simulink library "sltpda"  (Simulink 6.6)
InitFcn:
  | disp('Welcome to sLTPDA');
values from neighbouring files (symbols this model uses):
  filter = '*'    [uipickfiles.m]
  out = char(outs{j})    [sortCmds.m]    (also in uipickfiles.m = 0)
  param = params{get(handles.paramList, 'Value')}    [loopgui.m]
  plist = [plist cellstr(p.key)]    [sltpda_control.m]
undefined symbols (not defined in the file or in its folder): ao, chirp, foo_iir, Hanning, highpass, hist, Kaiser, linear, Normal, pole, pzmodel

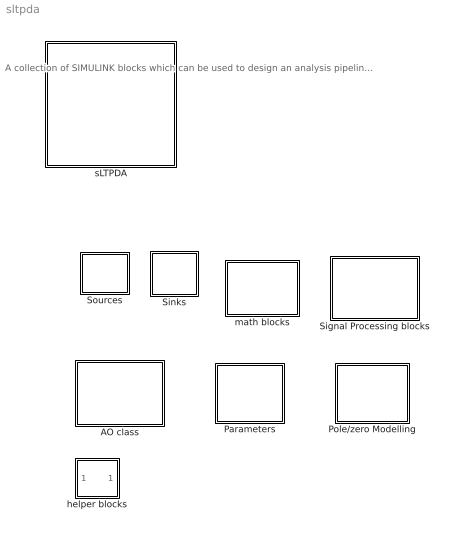
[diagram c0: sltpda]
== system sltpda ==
  note: A collection of SIMULINK blocks which can be used to design an analysis pipeline using LTPDA functions. The sLTPDA function set can be used to parse and run the model.
  AO class : Subsystem
  Parameters : Subsystem
  Pole/zero Modelling : Subsystem
  Signal Processing blocks : Subsystem
  Sinks : Subsystem
  Sources : Subsystem
  helper blocks : Subsystem
  math blocks : Subsystem
  sLTPDA : Subsystem

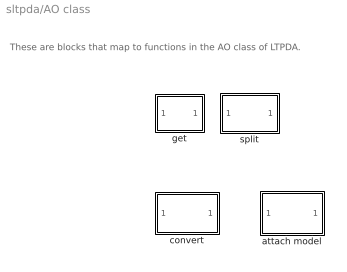
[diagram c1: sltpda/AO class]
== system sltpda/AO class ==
  note: These are blocks that map to functions in the AO class of LTPDA.
  attach model : Subsystem  Tag=attachdmdl
  convert : Subsystem  mask(convert){fcn=ao}
      mask prompts: fcn "convert to"
  get : Subsystem  Tag=get  Description=Get the propery of an analysis object.  mask(get){param=hist}
      mask prompts: param "parameter"
  split : Subsystem  Tag=split  Description=Splits an AO into many sub-AOs.  mask(split){method=times, splits=0}
      mask prompts: method "splitting method"

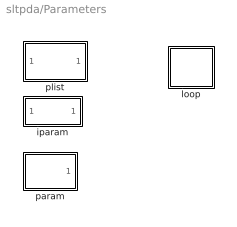
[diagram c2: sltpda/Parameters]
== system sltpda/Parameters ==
  iparam : Subsystem  Tag=iparam  mask(iparam){key=0}
      mask prompts: key "Parameter name"
  loop : Subsystem  mask(loop){block=<empty>, blockHandle=<empty>, key=0, vals=0, loopon=0, level=0}
      mask prompts: block "Block Name"; blockHandle "handle"; vals "values"
  param : Subsystem  Tag=param  mask(param){key=0, val=0}
      mask prompts: key "Parameter name"; val "Value"
  plist : Subsystem

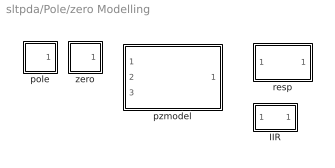
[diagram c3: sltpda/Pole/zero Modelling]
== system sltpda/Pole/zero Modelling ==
  IIR : Subsystem  mask(miir){fs=0}
      mask prompts: fs "Sample rate"
  pole : Subsystem  Tag=pole  mask(pole){polef=0, poleQ=0}
      mask prompts: polef "Frequency"; poleQ "Q"
  pzmodel : Subsystem
  resp : Subsystem  mask(resp){f1=, f2=, nf=, scale=linear}
      mask prompts: f1 "Start frequency"; f2 "Stop frequency"; nf "Number points"; scale "Sample spacing"
  zero : Subsystem  Tag=zero  mask(zero){zerof=0, zeroQ=0}
      mask prompts: zerof "Frequency"; zeroQ "Q"

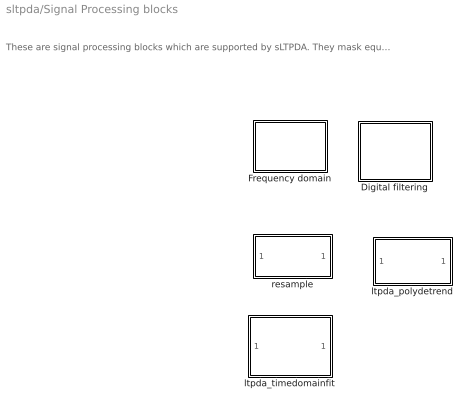
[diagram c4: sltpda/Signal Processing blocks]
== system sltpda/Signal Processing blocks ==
  note: These are signal processing blocks which are supported by sLTPDA. They mask equivalent functions which are in LTPDA.
  Digital filtering : Subsystem
  Frequency domain : Subsystem
  ltpda_polydetrend : Subsystem  Tag=ltpda_polydetrend  mask(ltpda_polydetrend){degree=1}
      mask prompts: degree "Degree of polynomial"
  ltpda_timedomainfit : Subsystem  Tag=ltpda_timedomainfit  Description=Performs a time-domain fit of the input AOs using ltpda_timedomainfit.
  resample : Subsystem  Tag=resample  mask(resample){fsout=0}
      mask prompts: fsout "Output sample rate"

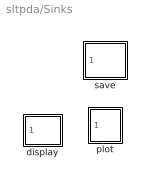
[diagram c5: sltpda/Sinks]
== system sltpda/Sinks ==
  display : Subsystem  Tag=display
  plot : Subsystem  Tag=plot  Description=Plot an analysis object.  mask(plot){xscale=linear, yscale=linear}
      mask prompts: xscale "x-scale"; yscale "y-scale"
  save : Subsystem  Tag=save  mask(save){fname=out.xml}
      mask prompts: fname "Filename"

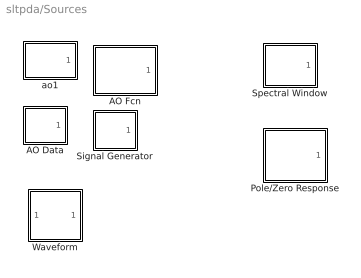
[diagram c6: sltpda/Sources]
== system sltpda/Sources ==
  AO Data : Subsystem  Tag=ao  mask(ao){vals=0}
      mask prompts: vals "data value(s)"
  AO Fcn : Subsystem  Tag=ao  mask(ao){fcn=0}
      mask prompts: fcn "Function"
  Pole/Zero Response : Subsystem  mask(pzmresp){pzm=pzmodel(plist([param('name', 'pzmodel') param('gain', [1]) param('poles', [ pole(plist([param('f', [1]) param('q', [0]) ]))]) param('zeros', []) ])), f1=0.1, f2=100, nf=1000}
      mask prompts: pzm "pzmodel constructor"; f1 "start frequency"; f2 "stop frequency"; nf "num points"
  Signal Generator : Subsystem  Tag=ao  mask(ao){nsecs=1, fs=100, tsfcn=sin(2*pi*10*t)}
      mask prompts: nsecs "Num seconds"; fs "Sample rate"; tsfcn "Function y(t)"
  Spectral Window : Subsystem  Tag=specwin  mask(specwin){wname=Hanning, wlen=1, psll=0}
      mask prompts: wname "Window type"; wlen "Length"
  Waveform : Subsystem  mask(ao){waveform=chirp, freq=0, phi=0, ntype=Normal, chirp_f0=0, chirp_fe=0, chirp_te=0, gp_f0=0, gp_bw=0, square_duty=0, sawtooth_width=0}
      mask prompts: freq "Frequency (Hz)"; phi "Phase offset [degrees]"; ntype "Noise type"; chirp_f0 "Start frequency (Hz)"; chirp_fe "Stop frequency (Hz)"; chirp_te "End time (s)"; gp_f0 "Central frequency (Hz)"; gp_bw "Bandwidth (Hz)"; square_duty "duty cycle [%]"; sawtooth_width "Width of sawtooth [0-1]"
  ao1 : Subsystem  Tag=ao  Description=Creates an Analysis object from a file.  mask(ao){fname=}
      mask prompts: fname "filename"

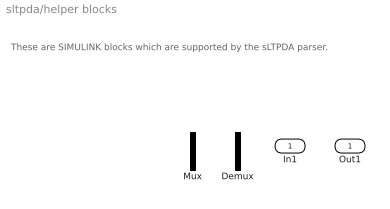
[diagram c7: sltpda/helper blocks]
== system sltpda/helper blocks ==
  note: These are SIMULINK blocks which are supported by the sLTPDA parser.
  In1 : Inport
  Demux : Demux  Outputs=2
  Mux : Mux  Inputs=2
  Out1 : Outport

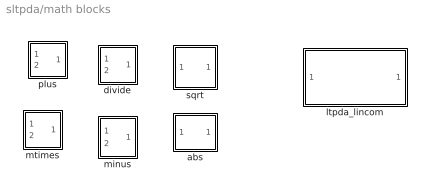
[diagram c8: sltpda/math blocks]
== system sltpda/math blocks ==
  abs : Subsystem
  divide : Subsystem  Tag=mrdivide
  ltpda_lincom : Subsystem  mask(ltpda_lincom){coeffs=0}
      mask prompts: coeffs "coefficients"
  minus : Subsystem  Tag=minus
  mtimes : Subsystem  Tag=mtimes
  plus : Subsystem  Tag=plus
  sqrt : Subsystem  Tag=sqrt

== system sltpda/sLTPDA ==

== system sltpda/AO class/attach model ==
  In1 : Inport
  Out1 : Outport

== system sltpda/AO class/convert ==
  In1 : Inport
  Out1 : Outport

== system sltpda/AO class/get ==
  ao in : Inport
  property out : Outport

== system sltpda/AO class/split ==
  In1 : Inport
  Out1 : Outport

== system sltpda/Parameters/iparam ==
  In1 : Inport
  Out1 : Outport

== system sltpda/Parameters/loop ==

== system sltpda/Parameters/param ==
  Out1 : Outport

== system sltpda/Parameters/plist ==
  In1 : Inport
  Out1 : Outport

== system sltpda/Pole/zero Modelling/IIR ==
  In1 : Inport
  Out1 : Outport

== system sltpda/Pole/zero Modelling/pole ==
  Out1 : Outport

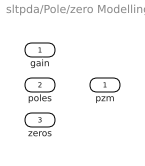
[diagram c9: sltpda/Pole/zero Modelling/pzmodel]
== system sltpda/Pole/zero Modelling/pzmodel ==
  gain : Inport
  poles : Inport  Port=2
  zeros : Inport  Port=3
  pzm : Outport

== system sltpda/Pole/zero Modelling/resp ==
  In1 : Inport
  Out1 : Outport

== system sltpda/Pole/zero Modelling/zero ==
  Out1 : Outport

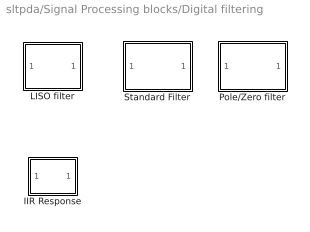
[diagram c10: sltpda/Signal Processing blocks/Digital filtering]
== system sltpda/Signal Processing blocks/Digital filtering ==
  IIR Response : Subsystem  mask(iirResp){f1=, f2=, nf=}
      mask prompts: f1 "Start Frequency"; f2 "Stop Frequency"; nf "Number points"
  LISO filter : Subsystem  Tag=filter  Description=Filter an AO.  mask(filter){fname=foo_iir.fil, method=filter}
      mask prompts: fname "filename"; method "filter method"
  Pole/Zero filter : Subsystem  mask(filter){method=filter, miirstr=pzmodel(plist([param('name', 'pzmodel') param('gain', [1]) param('poles', [ pole(plist([param('f', [1]) param('q', [0]) ]))]) param('zeros', []) ]))}
      mask prompts: method "filter method"; miirstr "constructor string"
      mask help: Filter using an IIR filter based on a pole/zero design. Use pzmodel_helper GUI to create the miir constructor string.
  Standard Filter : Subsystem  Tag=filter  Description=Apply a standard filter type to input AO.  mask(filter){method=filter, ftype=highpass, fgain=1, ffc=0.5, forder=1}
      mask prompts: ftype "filter type"; fgain "gain"; ffc "corner frequencie(s) [Hz]"; forder "filter order"

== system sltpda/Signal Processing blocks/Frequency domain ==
  ltpda_lpsd : Subsystem  Tag=ltpda_psd  mask(ltpda_lpsd){Kdes=100, Kmin=1, Jdes=100, win=Kaiser, psll=100, olap=0}
      mask prompts: Kdes "Desired num averages"; Kmin "Minimum num averages"; Jdes "Number of spectral frequencies"; win "Window"; olap "Overlap"
  ltpda_pwelch : Subsystem  Tag=ltpda_pwelch  Description=Makes a spectral density estimate by calling ltpda_pwlech.  mask(ltpda_pwelch){Nfft=, Nolap=}
      mask prompts: Nfft "Num points in FFT"; Nolap "Overlap (samples)"
  ltpda_tfe : Subsystem  Tag=ltpda_tfe  Description=Calls ltpda_tfe.  mask(ltpda_tfe){win=Hanning, nfft=, psll=, nolap=}
      mask prompts: win "Window"; nolap "Overlap (samples)"
      mask help: Computes a transfer function estimate given the input and output of the system. This calls ltpda_tfe() which in turn calls tfestimate().

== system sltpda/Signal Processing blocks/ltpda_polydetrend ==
  In1 : Inport
  Out1 : Outport

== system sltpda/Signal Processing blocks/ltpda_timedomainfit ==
  In1 : Inport
  Out1 : Outport

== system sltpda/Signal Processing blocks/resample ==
  In1 : Inport
  Out1 : Outport

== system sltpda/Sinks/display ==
  In1 : Inport

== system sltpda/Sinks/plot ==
  ao in : Inport

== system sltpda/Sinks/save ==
  In1 : Inport

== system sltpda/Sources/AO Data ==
  Out1 : Outport

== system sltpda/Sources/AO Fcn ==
  Out1 : Outport

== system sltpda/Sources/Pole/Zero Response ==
  Out1 : Outport

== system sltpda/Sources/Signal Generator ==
  Out1 : Outport

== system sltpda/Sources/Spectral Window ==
  Out1 : Outport

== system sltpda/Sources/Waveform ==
  pl : Inport
  Out1 : Outport

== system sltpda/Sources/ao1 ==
  out : Outport

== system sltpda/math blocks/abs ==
  In1 : Inport
  Out1 : Outport

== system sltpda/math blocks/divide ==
  In3 : Inport
  In4 : Inport  Port=2
  Out2 : Outport

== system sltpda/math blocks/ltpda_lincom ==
  In1 : Inport
  Out1 : Outport

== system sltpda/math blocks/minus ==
  In3 : Inport
  In4 : Inport  Port=2
  Out2 : Outport

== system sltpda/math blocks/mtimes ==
  In3 : Inport
  In4 : Inport  Port=2
  Out2 : Outport

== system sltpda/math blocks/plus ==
  In1 : Inport
  In2 : Inport  Port=2
  Out1 : Outport

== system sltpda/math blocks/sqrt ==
  In1 : Inport
  Out1 : Outport

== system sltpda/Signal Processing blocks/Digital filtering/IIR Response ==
  In1 : Inport
  Out1 : Outport

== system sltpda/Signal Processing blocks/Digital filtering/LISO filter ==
  ao in : Inport
  property out : Outport

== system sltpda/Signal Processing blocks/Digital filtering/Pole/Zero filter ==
  In1 : Inport
  Out1 : Outport

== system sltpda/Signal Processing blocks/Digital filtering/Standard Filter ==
  In1 : Inport
  Out1 : Outport

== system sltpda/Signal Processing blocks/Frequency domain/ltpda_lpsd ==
  In1 : Inport
  Out1 : Outport

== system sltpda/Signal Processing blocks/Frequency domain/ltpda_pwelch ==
  In1 : Inport
  pl : Inport  Port=2
  Out1 : Outport

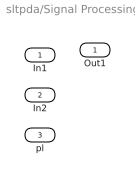
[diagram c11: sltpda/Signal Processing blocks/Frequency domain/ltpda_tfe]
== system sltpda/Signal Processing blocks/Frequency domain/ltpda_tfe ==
  In1 : Inport
  In2 : Inport  Port=2
  pl : Inport  Port=3
  Out1 : Outport
